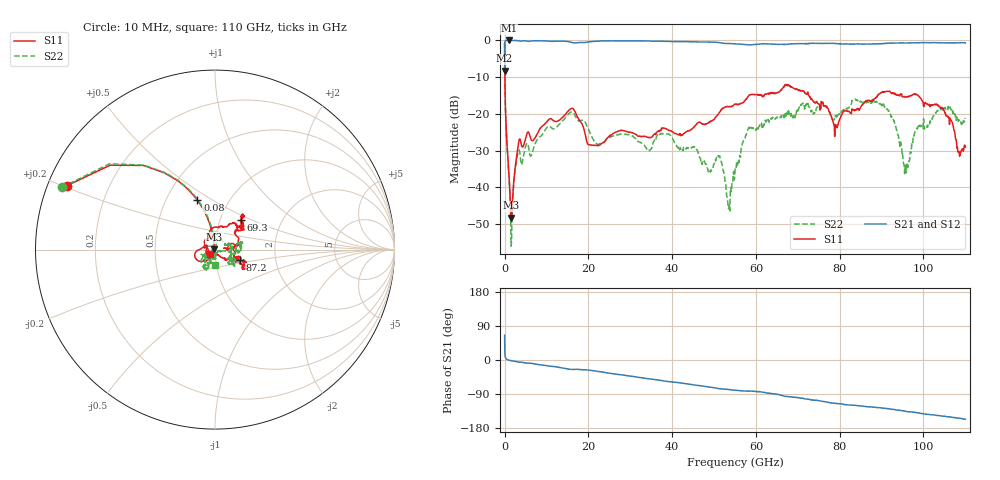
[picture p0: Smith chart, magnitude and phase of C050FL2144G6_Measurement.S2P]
! Data measured by Modelithics Inc.  support@modelithics.com  813-866-6335  Tampa FL USA June 2025
! PPI-050FL-0R28-280-G6_0p28uH measured on 5-mil thick RO3003G2 board, mounted in 2-port shunt configuration on a 50-ohm transmission line
# GHz S RI R 50.0
!freq ReS11 ImS11 ReS21 ImS21 ReS12 ImS12 ReS22 ImS22
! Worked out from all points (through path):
!   1207 points, 10 MHz to 110 GHz, reference 50 ohm
!   highest |S21| = -0.04 dB at 979.6 MHz (marker M1); lowest = -8.3 dB at 10 MHz (marker M2)
!   group delay of S21, straight-line fit = 3.98 ps
!   lowest |S11| = -48.3 dB at 1.562 GHz (marker M3), VSWR 1.01, Z = 49.6 + j0.0964 ohm
!   |S11| at or under -10 dB: 73.09 MHz to end of sweep
!   |S22| runs from -56.0 to -0.7 dB; largest |S21 - S12| = 0.082
!   S11 on the Smith chart (normalised r, x): 10 MHz: 0.06, +0.21; 80 MHz: 0.71, +0.43; 69.3 GHz: 1.25, +0.43; 87.2 GHz: 1.31, -0.15; 110 GHz: 0.95, -0.04
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0.01  -0.8258 0.3557  0.1604 0.352  0.1603 0.3519  -0.8543 0.3468
0.08  -0.0981 0.2746  0.9038 0.2734  0.9038 0.2734  -0.0946 0.276
0.2  -0.0224 0.1206  0.9793 0.1165  0.9793 0.1165  -0.0189 0.1213
0.9796215  -0.00443 0.0168  0.9956 -0.00316  0.9955 -0.00294  -0.00119 0.0168
1.562154  -0.00373 0.000972  0.9951 -0.0298  0.9951 -0.0294  -0.00128 0.000925
3.018486  -0.00671 -0.0293  0.9873 -0.0864  0.9874 -0.0854  -0.0102 -0.0243
5.445706  -0.0329 -0.0446  0.9623 -0.1442  0.9625 -0.1429  -0.0246 -0.0312
18.35852  -0.0748 0.00725  0.8421 -0.4021  0.8421 -0.4022  -0.0643 -0.0496
21.077  -0.0353 -0.0124  0.8511 -0.4524  0.8512 -0.4523  -0.0404 -0.0217
36.7083  -0.0552 0.0198  0.5874 -0.7783  0.5844 -0.7805  0.00336 -0.0529
51.17453  -0.0306 0.0975  0.2372 -0.9  0.2327 -0.9012  -0.0154 -0.0213
53.50466  0.0125 0.124  0.1903 -0.8842  0.1983 -0.8825  -0.00081 0.00506
55.05808  0.0355 0.1304  0.1571 -0.8795  0.164 -0.878  0.00313 0.0176
58.45619  0.0994 0.1501  0.1211 -0.8595  0.1107 -0.861  0.0428 0.0444
69.3  0.1447 0.1648  -0.1328 -0.8894  -0.1093 -0.8913  0.0769 -0.0439
73.4  0.1128 0.1067  -0.2481 -0.8743  -0.1868 -0.8862  0.0739 -0.0733
79.1  0.0709 -0.00203  -0.375 -0.8227  -0.3269 -0.8412  0.0934 0.0177
87.2  0.1377 -0.0562  -0.4948 -0.7412  -0.4618 -0.7627  0.1401 0.0329
91.7  0.1721 -0.1055  -0.5657 -0.7169  -0.5696 -0.7197  0.1083 -0.0228
95.8  0.1589 -0.0619  -0.6582 -0.6435  -0.6397 -0.6647  0.0143 -0.00953
103.4  0.1196 -0.0592  -0.7737 -0.5104  -0.7582 -0.5315  -0.0585 -0.0926
110  -0.0268 -0.023  -0.8462 -0.3686  -0.8481 -0.3737  0.00266 -0.0876
